FUNCTION_BLOCK FB_MachineData_BIN
VAR_INPUT
	bRunOnCeDevice				: BOOL	:= TRUE;	(*在CE系统运行*)
	sgFilePath					: STRING(255)	:= 'Data\Machine\';	(*文件路径*)
	sgFileName					: STRING(255)	:= 'Test';			(*文件名*)
(*参数和备份(用来比较参数是否修改的)的类型必须一致, 把两个变量的首地址和数据长度传到功能块*)
	pMacData					: PVOID;			(*配方首地址*)
	pBakData					: PVOID;			(*配方备份数据首地址, 数据类型必须和配方一样*)
	nMacSize					: UDINT;			(*配方的字节数*)
	tAutoSave					: TIME	:= T#10S;	(*配方改变后, 延时保存*)
END_VAR
VAR_OUTPUT
(*状态*)
	bInitialDone				: BOOL;	(*初始化完成*)
	bDone						: BOOL;
	bBusy						: BOOL;
	bError						: BOOL;
END_VAR
VAR		
	eStep						: INT;
(*Last status*)
	s_sLastExecuteResult		: ST_LastExecutionResult_File;
(*FB*)
	s_fbWriteReadFile			: FB_WriteReadFileBIN_2;
	s_nErrorCounter				: UDINT;
(*参数改变, 延时触发写文件*)
	s_tonDataChange				: TON;
	s_bDataChange				: BOOL;
	s_bManualWriteOnce			: BOOL;
END_VAR

(*==================================================================
配置
==================================================================*)
	s_tonDataChange.PT					:= tAutoSave;		(*参数修改后, 延时写入临时文件(作用是掉电保持)的时间*)


(*==================================================================
变量地址是否有误
==================================================================*)
IF pMacData = 0 OR nMacSize <= 0 OR pBakData = 0 THEN
	bInitialDone := bBusy := bDone := FALSE;
	eStep := 0;
	bError := TRUE;
	RETURN;
END_IF


(*==================================================================
判断参数是否变化, 变化后, 延时写入文件
==================================================================*)
(*参数比较, 有变化时, 延时置位s_bDataChange, 将当前参数写到临时文件中*)
IF pMacData <> 0 AND nMacSize > 0 AND pBakData <> 0 THEN
	IF MEMCMP(pBakData, pMacData, nMacSize) <> 0 THEN
		s_tonDataChange(IN := FALSE);		(*重新计时*)
		s_tonDataChange(IN := bInitialDone);	(*上载配方后, 只复制参数, 不写入临时文件*)
		MEMCPY(pBakData, pMacData, nMacSize);	(*比较不同, 重新定时, 并把数据复制到局部变量*)
	END_IF
ELSE
	bInitialDone := FALSE;
END_IF

s_tonDataChange();

s_bDataChange := FALSE;
IF s_tonDataChange.Q THEN
	s_tonDataChange(IN := FALSE);
	s_bDataChange := TRUE;
END_IF


(*保存路径*)
IF bRunOnCeDevice THEN
	s_fbWriteReadFile.sgDeviceName	:= '\Hard disk\';
ELSE
	s_fbWriteReadFile.sgDeviceName	:= 'C:\';
END_IF
	s_fbWriteReadFile.sgFolderName	:= sgFilePath;
	s_fbWriteReadFile.sgNetId		:= '';
	s_fbWriteReadFile.sOption.bSameAddress_RW		:= FALSE;
	s_fbWriteReadFile.sOption.sBinHeader.bInused	:= FALSE;


(*读写流程*)
CASE eStep OF
	0:
		bDone := bError := FALSE;
		IF NOT bInitialDone THEN
			MEMSET(ADR(s_sLastExecuteResult), 0, SIZEOF(s_sLastExecuteResult));
			s_fbWriteReadFile(bReadFile := FALSE, bWriteFile := FALSE);
			eStep := 100;
		ELSE
			IF s_bDataChange					(*数据变化后, 延时写入*)
			OR s_bManualWriteOnce THEN			(*手动写入一次(测试用)*)
				MEMSET(ADR(s_sLastExecuteResult), 0, SIZEOF(s_sLastExecuteResult));
				s_bDataChange := FALSE;
				s_bManualWriteOnce := FALSE;
				s_fbWriteReadFile(bReadFile := FALSE, bWriteFile := FALSE);
				eStep := 200;
			END_IF
		END_IF

	100:	(*读取文件, 循环, 一直判断是否需要读取, 知道最大数量*)
		s_fbWriteReadFile.pDestBuffer	:= pMacData;
		s_fbWriteReadFile.u32DestSize	:= nMacSize;
		s_fbWriteReadFile.sgFileName	:= sgFileName;
		s_fbWriteReadFile(bReadFile := TRUE);
		s_nErrorCounter					:= 0;
		eStep := 150;
	150:
		s_fbWriteReadFile(bReadFile := TRUE);
		IF NOT s_fbWriteReadFile.bBusy THEN
			IF NOT s_fbWriteReadFile.bError THEN
				MEMCPY(pBakData, pMacData, nMacSize);	(*读取完, 把值传给中间变量*)
				bDone := TRUE;
				eStep := 0;
			ELSE
				s_nErrorCounter := s_nErrorCounter + 1;	(*连续读写失败, 可能是文件不存在, 跳过*)
				IF s_nErrorCounter > 5 THEN
					bError := TRUE;
					eStep := 0;
				END_IF
			END_IF
			s_bDataChange := FALSE;
			s_bManualWriteOnce := FALSE;
			s_fbWriteReadFile(bReadFile := FALSE, bWriteFile := FALSE);
		END_IF
	200:
		s_fbWriteReadFile.pSrcBuffer	:= pMacData;
		s_fbWriteReadFile.u32SrcSize	:= nMacSize;
		s_fbWriteReadFile.sgFileName	:= sgFileName;
		s_fbWriteReadFile(bWriteFile := TRUE);
		eStep := 250;
	250:
		s_fbWriteReadFile(bWriteFile := TRUE);
		IF s_fbWriteReadFile.bWriteFile THEN
			s_fbWriteReadFile(bWriteFile := TRUE);
			IF NOT s_fbWriteReadFile.bBusy THEN
				IF NOT s_fbWriteReadFile.bError THEN
					bDone := TRUE;
				ELSE
					bError := TRUE;
				END_IF
				s_fbWriteReadFile(bReadFile := FALSE, bWriteFile := FALSE);
				eStep := 0;
			END_IF
		END_IF
END_CASE


IF eStep <> 0 THEN
	bBusy := TRUE;
ELSE
	IF bBusy THEN
		bBusy := FALSE;
		bInitialDone := TRUE;			(*不管有没有读取成功, 都认为初始化完成*)
		s_sLastExecuteResult.bDone := bDone;
		s_sLastExecuteResult.bError := bError;
	END_IF
END_IF

END_FUNCTION_BLOCK
